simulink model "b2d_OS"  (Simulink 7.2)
settings: Solver=ode3  SolverMode=SingleTasking  StartTime=0.0  StopTime=0.2  FixedStep=10e-6  MaxStep=1e-5  RelTol=1e-3  AbsTol=1e-3

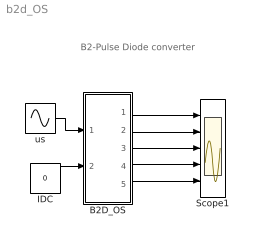
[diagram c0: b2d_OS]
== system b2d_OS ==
  note: B2-Pulse Diode converter
  B2D_OS : Subsystem  mask(b2d_OS){LS=1e-3, LD=1e-3, ILD0=80, C=1e-5, VC0=80, RD=2}
      mask prompts: LS "Source Inductance"; LD "Load Inductance"; ILD0 "initial  Load Inductance Current"; C "Load Cap"; VC0 "initial Cap Voltage"; RD "Load Resistance"
      mask help: Open Source 2-Pulse Diode Bridge Converter Input Vector u: u[0]= Vs.v u[1]= IDC.i Output Vector y: y[0]= D1.I y[1]= D1.V y[2]= Lc.I y[3]= Ld.I y[4]= VDC.V y[5]= VC.V Parameter Vector p: p[0]= Lc.L p[1]= Ld.L p[2]= Ld.IL0 p[3]= C1.C p[4]= C1.vC0 p[5]= R1.r You can pause the simulation during running, change the Parameters you want and continue the Simulation
  IDC : Constant  Value=0  OutDataType=sfix(16)  OutScaling=2^0
  Scope1 : Scope  NumInputPorts=5
  us : Sin  Amplitude=230*sqrt(2)  Frequency=2*pi*50  SampleTime=0
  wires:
  us/1 -> B2D_OS/1(vS)
  IDC/1 -> B2D_OS/2(iDC)
  B2D_OS/1(iD1,vD1) -> Scope1/1
  B2D_OS/2(iLc) -> Scope1/2
  B2D_OS/3(iLd) -> Scope1/3
  B2D_OS/4(vDC) -> Scope1/4
  B2D_OS/5(vC) -> Scope1/5

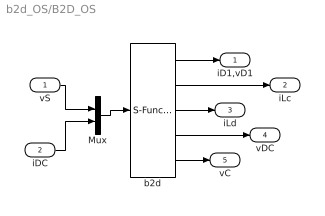
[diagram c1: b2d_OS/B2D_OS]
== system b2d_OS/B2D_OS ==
  vS : Inport  OutDataType=sfix(16)  OutScaling=2^0
  iDC : Inport  Port=2  OutDataType=sfix(16)  OutScaling=2^0
  Mux : Mux  Inputs=2
  b2d : S-Function  FunctionName=s_b2d_OS  Parameters="[ LS LD  ILD0  C  VC0 RD]"  EnableBusSupport=off
  iD1,vD1 : Outport  OutDataType=sfix(16)  OutScaling=2^0
  iLc : Outport  Port=2  OutDataType=sfix(16)  OutScaling=2^0
  iLd : Outport  Port=3  OutDataType=sfix(16)  OutScaling=2^0
  vDC : Outport  Port=4  OutDataType=sfix(16)  OutScaling=2^0
  vC : Outport  Port=5  OutDataType=sfix(16)  OutScaling=2^0
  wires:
  b2d/1 -> iD1,vD1/1
  b2d/2 -> iLc/1
  vS/1 -> Mux/1
  iDC/1 -> Mux/2
  Mux/1 -> b2d/1
  b2d/3 -> iLd/1
  b2d/4 -> vDC/1
  b2d/5 -> vC/1
